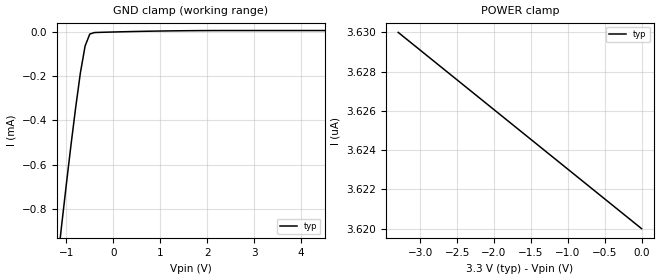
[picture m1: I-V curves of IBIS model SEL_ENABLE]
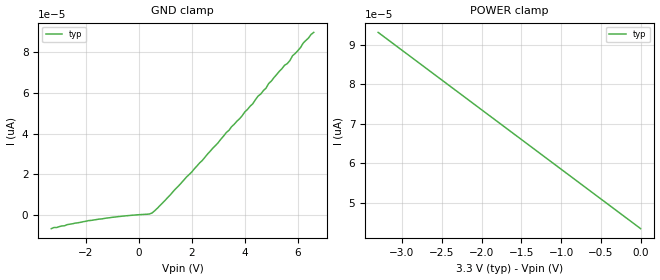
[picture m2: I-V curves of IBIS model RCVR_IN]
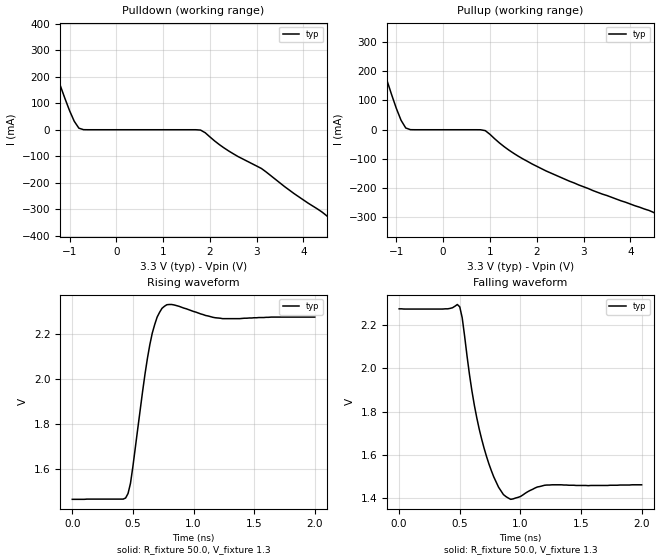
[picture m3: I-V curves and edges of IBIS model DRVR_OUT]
|   Texas Instruments Incorporated
|   Data Transmissions Products
|   IBIS Model for SN65LVCP23
|   16D SOIC Package
[IBIS Ver]   3.2
[Comment char]   |_char
[File name]   lvcp23.ibs
[File Rev]   2.0
[Date]   10Jun03
[Source]   File originated at Texas Instruments Incorporated.
   Data Transmission Products Group.
[Notes]
[Disclaimer]
(C) Copyright Texas Instruments Incorporated 2003
   All rights reserved
  Texas Instruments Incorporated hereby grants the user of this IBIS
model a non-exclusive, nontransferable license to use this IBIS model
under the following terms.  Before using this IBIS model, the user
should read this license.  If the user does not accept these terms,
the IBIS model should be returned to Texas Instruments within 30 days.
  The user is granted this license only to use the IBIS model and
is not granted rights to sell, load, rent, lease or license the IBIS
model in whole or in part, or in modified form to anyone other than
user.  User may modify the IBIS model to suit its specific applications
but rights to derivative works and such modifications shall belong to
Texas Instruments.
  This IBIS model is provided on an "AS IS" basis and Texas Instruments
makes absolutely no warranty with respect to the information contained
herein.  TEXAS INSTRUMENTS DISCLAIMS AND CUSTOMER WAIVES ALL WARRANTIES,
EXPRESS OR IMPLIED, INCLUDING WARRANTIES OF MERCHANTABILITY OR FITNESS
FOR A PARTICULAR PURPOSE. The entire risk as to quality and performance
is with the Customer. ACCORDINGLY, IN NO EVENT SHALL THE COMPANY BE LIABLE
FOR ANY DAMAGES, WHETHER IN CONTRACT OR TORT,INCLUDING ANY LOST PROFITS
OR OTHER INCIDENTAL, CONSEQUENTIAL, EXEMPLARY, OR PUNITIVE DAMAGES ARISING
OUT OF THE USE OR APPLICATION OF THE IBIS model provided in this package.
Further, Texas Instruments reserves the right to discontinue or make changes
without notice to any product herein to improve reliability, function, or
design. Texas Instruments does not convey any license under patent rights
or any other intellectual property rights, including those of third parties.
Contact Texas Instruments at ATTN:DATA TRANSMISSIONS
[Copyright]   Copyright 2003, Texas Instruments, All Rights Reserved
[Component]   LVCP23D
[Manufacturer]  Texas Instruments Incorporated
[Package]
|   typ   min   max
R_pkg   0.035   0.030   0.040
L_pkg   2.181nH   1.231nH   3.257nH
C_pkg   0.322pF   0.163pF   0.546pF
[Pin]   signal_name   model_name   R_pin   L_pin   C_pin
1   SEL1   SEL_ENABLE   0.040   3.251n   0.546p
2   SEL0   SEL_ENABLE   0.039   2.561n   0.393p
3   INO+   RCVR_IN   0.030   1.681n   0.186p
4   INO-   RCVR_IN   0.030   1.231n   0.163p
5   VCC   POWER   0.030   1.231n   0.163p
6   IN1+   RCVR_IN   0.030   1.681n   0.186p
7   IN1-   RCVR_IN   0.039   2.564n   0.393p
8   NC   NC
9   NC   NC
10   OUT1-   DRVR_OUT   0.039   2.558n   0.394p
11   OUT1+   DRVR_OUT   0.030   1.681n   0.187p
12   GND   GND   0.030   1.231n   0.163p
13   OUT0-   DRVR_OUT   0.030   1.231n   0.163p
14   OUT0+   DRVR_OUT   0.030   1.681n   0.187p
15   EN1   SEL_ENABLE   0.039   2.558n   0.394p
16   EN0   SEL_ENABLE   0.040   3.246n   0.546p
[Diff_pin]   inv_pin   vdiff   tdelay_typ   tdelay_min   tdelay_max
| The 'xY' pin is Diff_pin and the 'xZ' pin is the inv_pin
3   4   0.100   0 0 0
6   7   0.100   0 0 0
11   10   NA   0 0 0
14   13   NA   0 0 0
| Models and submodels in the file (3): SEL_ENABLE (Input), RCVR_IN (Input), DRVR_OUT (Output_ECL)
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|   Select/Enable Model
[Model]   SEL_ENABLE
Model_type   Input
|Signals   SEL0,SEL1,EN0,EN1
Vinh = 2.0
Vinl = 0.8
|   typ   min   max
C_comp   1.27pF   NA   NA
|   typ   min   max
[Temperature Range]   25.0   NA   NA
[Voltage range]   3.3V   3.0V   3.6V
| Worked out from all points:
|   GND clamp passes 1 mA (typ) near -1.16 V on its own axis
[GND_clamp]
|Voltage  I(typ)   I(min)   I(max)
-3.3V     -6.29mA    NA         NA
-1.2V     -1.07mA    NA         NA
-1.1V     -876uA     NA         NA
-900mV    -511uA     NA         NA
-800mV    -341uA     NA         NA
-700mV    -185uA     NA         NA
-600mV    -63.8uA    NA         NA
-500mV    -9.29uA    NA         NA
-400mV    -2.58uA    NA         NA
-300mV    -1.78uA    NA         NA
1.4V      5.48uA     NA         NA
6.6V      6.65uA     NA         NA
[Power_clamp]
| Note that the[POWER_clamp]voltage table is referenced to Vcc
| and is calculated using Vtable=Vcc - Vmeasured.
|Voltage  I(typ)   I(min)   I(max)
-3.3V     3.63uA     NA         NA
0V        3.62uA     NA         NA
|   Receiver Input Model
[Model]   RCVR_IN
Model_type   Input
|Signals   IN0+,IN0-,IN1+,IN1-
Vinh = 1.4
Vinl = 1.0
|   typ   min   max
C_comp   1.16pF   NA   NA
|   typ   min   max
[Temperature Range]   25.0   NA   NA
[Voltage range]   3.3V   3.0V   3.6V
[GND_clamp]
|Voltage  I(typ)   I(min)   I(max)
-3.3V     -6.87pA    NA         NA
-1.9V     -2.91pA    NA         NA
500mV     849fA      NA         NA
2.4V      26.8pA     NA         NA
4.3V      54.7pA     NA         NA
4.8V      62.4pA     NA         NA
4.9V      64.7pA     NA         NA
5.7V      76pA       NA         NA
5.8V      78.4pA     NA         NA
6.1V      82.4pA     NA         NA
6.2V      84.6pA     NA         NA
6.6V      89.9pA     NA         NA
[Power_clamp]
| Note that the[POWER_clamp]voltage table is referenced to Vcc
| and is calculated using Vtable=Vcc - Vmeasured.
|Voltage  I(typ)   I(min)   I(max)
-3.3V     93.1pA     NA         NA
0V        43.4pA     NA         NA
|   Driver Output Model
[Model]   DRVR_OUT
Model_type   Output_ECL
| Signals   OUT0+,OUT0-,OUT1+,OUT1-
Vmeas = 2.0V   |Reference voltage for timing measurements
Cref = 1pF   |Timing specification test load capacitance value
Rref = 50
|Note: 50 Ohm load; single ended configuration
| variable   typ   min   max
C_comp   1.60pF   NA   NA
|   typ   min   max
[Temperature Range]   25.0   NA   NA
[Voltage range]   3.3V   3.0V   3.6V
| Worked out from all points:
|   rising waveform, R_fixture 50.0, V_fixture 1.3: 20-80 % time 123ps typ, NA min, NA max; typ from 1.46 V to 2.27 V
|   falling waveform, R_fixture 50.0, V_fixture 1.3: 20-80 % time 156ps typ, NA min, NA max; typ from 2.27 V to 1.46 V
[Pulldown]
|Voltage  I(typ)   I(min)  I(max)
| Note that the [Pulldown] voltage table is referenced to Vcc
| and is calculated using Vtable=Vcc - Vmeasured.
-3.3V     1.47A      NA         NA
-1.6V     385mA      NA         NA
-1.1V     119mA      NA         NA
-900mV    32.3mA     NA         NA
-800mV    5.95mA     NA         NA
1.8V      -1.24mA    NA         NA
2.4V      -79.9mA    NA         NA
3.1V      -146mA     NA         NA
3.8V      -241mA     NA         NA
4.4V      -311mA     NA         NA
4.8V      -384mA     NA         NA
6.6V      -587mA     NA         NA
[Pullup]
|   Voltage   I(typ)   I(min)   I(max)
| Note that the[Pullup]voltage table is referenced to Vcc
| and is calculated using Vtable=Vcc - Vmeasured.
-3.3V     1.47A      NA         NA
-1.6V     385mA      NA         NA
-1.5V     328mA      NA         NA
-1V       72.5mA     NA         NA
-800mV    5.95mA     NA         NA
900mV     -3.08mA    NA         NA
1.4V      -69.2mA    NA         NA
1.9V      -117mA     NA         NA
2.9V      -189mA     NA         NA
4.5V      -283mA     NA         NA
5V        -349mA     NA         NA
6.6V      -540mA     NA         NA
[Ramp]
|   typ   min   max
dV/dt_r   0.585/130ps   NA   NA
dV/dt_f   0.585/170ps   NA   NA
R_load = 50ohm  |Note: The measurement is with 50ohm to Vtt.
[Rising Waveform]
R_fixture = 50.0
V_fixture = 1.3
V_fixture_min = 1.0
V_fixture_max = 1.6
C_fixture = 0p
L_fixture = 0n
|   V(typ)  V(min)  V(max)
0s        1.464V     NA         NA
420ps     1.465V     NA         NA
460ps     1.49V      NA         NA
480ps     1.535V     NA         NA
600ps     2.022V     NA         NA
640ps     2.153V     NA         NA
700ps     2.275V     NA         NA
760ps     2.323V     NA         NA
1.24ns    2.268V     NA         NA
2ns       2.275V     NA         NA
[Falling Waveform]
R_fixture = 50.0
V_fixture = 1.3
V_fixture_min = 1.0
V_fixture_max = 1.6
C_fixture = 0p
L_fixture = 0n
|   V(typ)  V(min)  V(max)
0s        2.275V     NA         NA
500ps     2.284V     NA         NA
520ps     2.234V     NA         NA
600ps     1.897V     NA         NA
660ps     1.721V     NA         NA
780ps     1.5V       NA         NA
880ps     1.409V     NA         NA
940ps     1.398V     NA         NA
1.22ns    1.462V     NA         NA
2ns       1.463V     NA         NA
